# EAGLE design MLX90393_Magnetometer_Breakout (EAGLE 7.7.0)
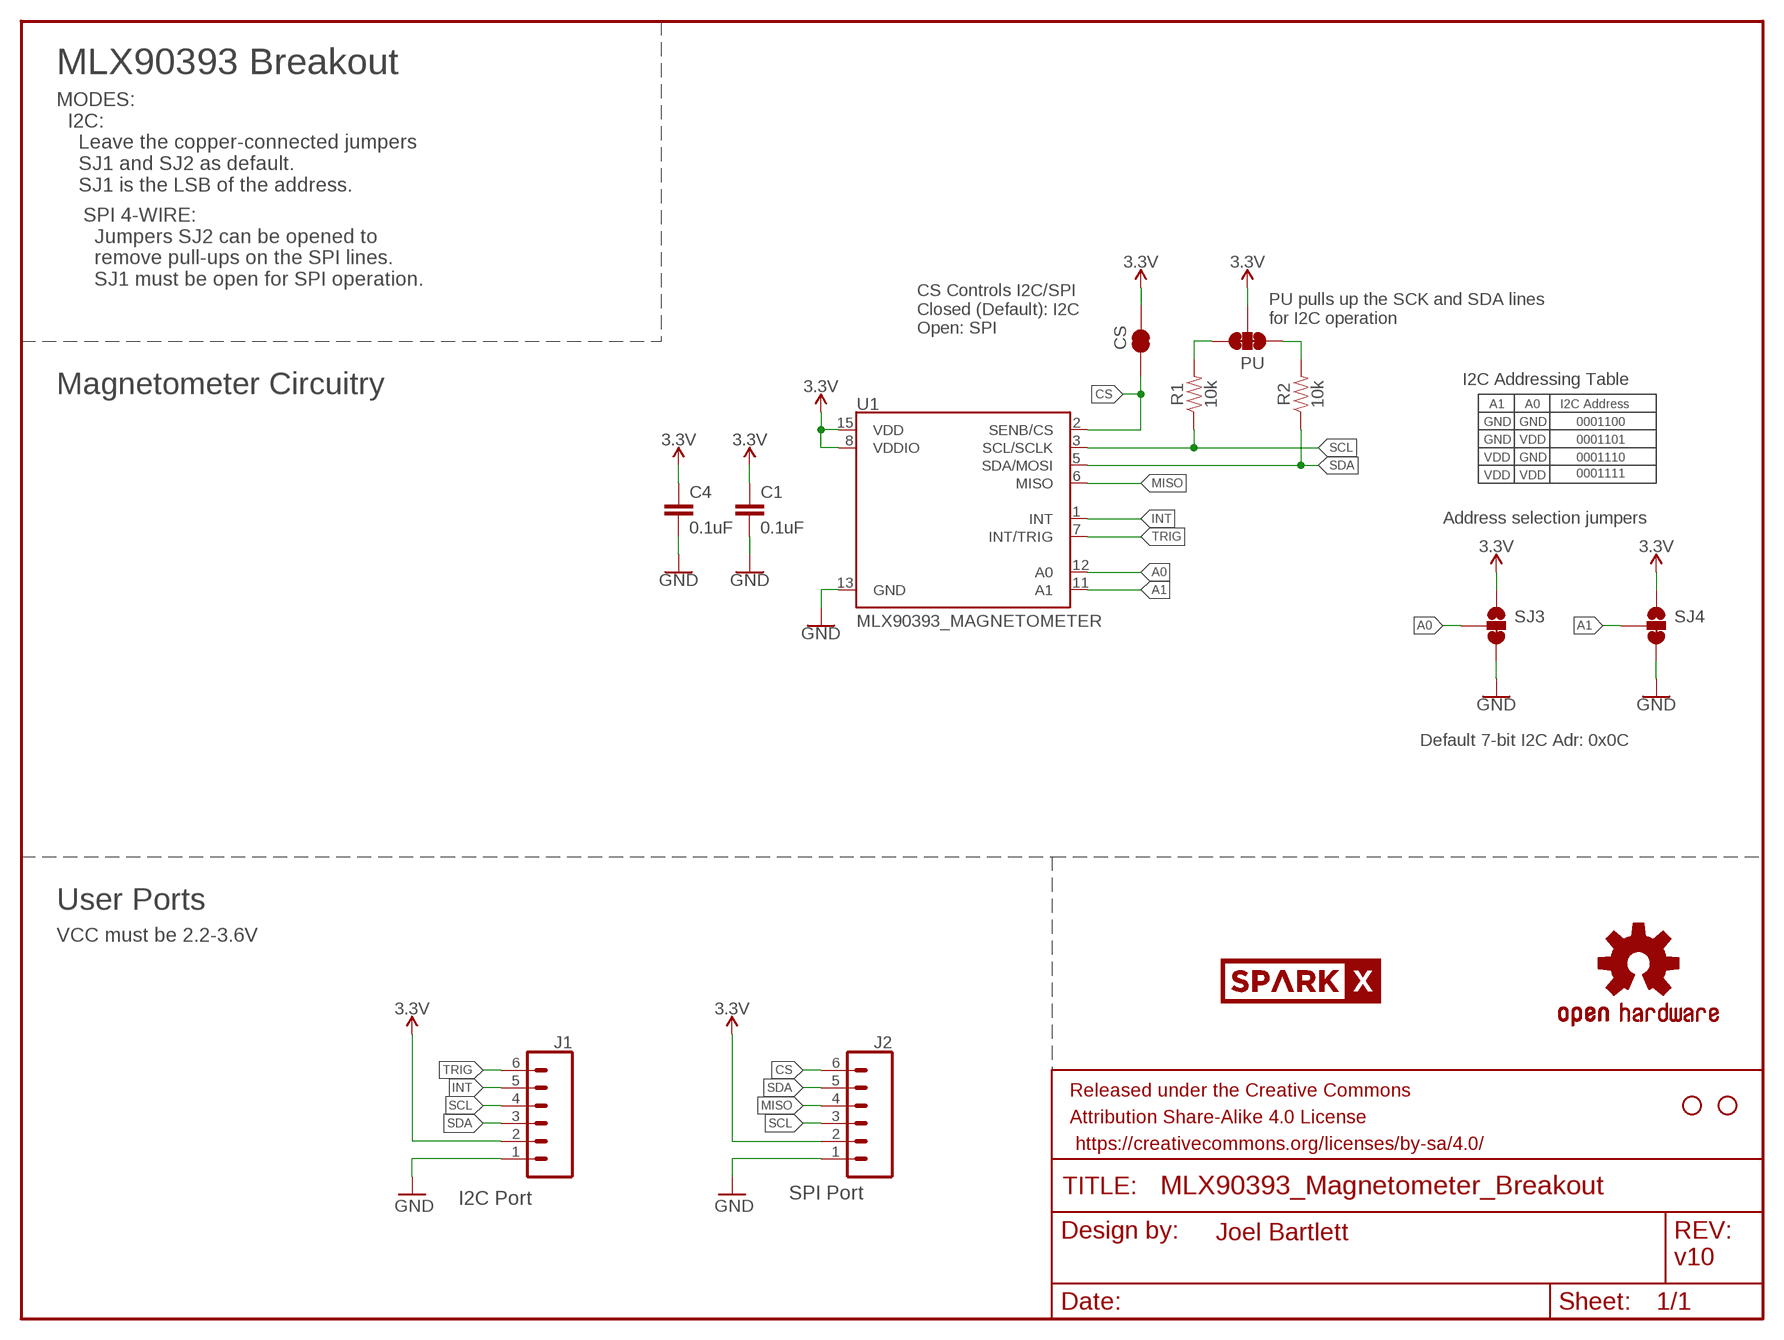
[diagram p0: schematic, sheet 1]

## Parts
C1  0.1uF  0.1UF-0603-25V-(+80/-20%)  [0603]
C4  0.1uF  0.1UF-0603-25V-(+80/-20%)  [0603]
CS  JUMPER-SMT_2_NC_TRACE_SILK  [SMT-JUMPER_2_NC_TRACE_SILK]
FRAME2  FRAME-LETTER  [CREATIVE_COMMONS]
J1  CONN_06NO_SILK_FEMALE_PTH  [1X06_NO_SILK]
J2  CONN_06NO_SILK_FEMALE_PTH  [1X06_NO_SILK]
JP3  STAND-OFF  [STAND-OFF]
JP4  STAND-OFF  [STAND-OFF]
PU  JUMPER-PAD-3-NC_BY_TRACE  [PAD-JUMPER-3-3OF3_NC_BY_TRACE_YES_SILK_FULL_BOX]
R1  10k  10KOHM-0603-1/10W-1%  [0603]
R2  10k  10KOHM-0603-1/10W-1%  [0603]
SJ3  JUMPER-SMT_3_1-NC_TRACE_SILK  [SMT-JUMPER_3_1-NC_TRACE_SILK]
SJ4  JUMPER-SMT_3_1-NC_TRACE_SILK  [SMT-JUMPER_3_1-NC_TRACE_SILK]
U1  MLX90393_MAGNETOMETER  [QFN-16]
U$1  OSHW-LOGOS  [OSHW-LOGO-S]
U$2  SPARKX-LOGO2  [SPARKX-TINY]

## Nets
3.3V: C1.1 C4.1 CS.2 J1.2 J2.2 PU.2 SJ3.1 SJ4.1 U1.8(VDDIO) U1.15(VDD)
A0: SJ3.2 U1.12(A0)
A1: SJ4.2 U1.11(A1)
CS: CS.1 J2.6 U1.2(SENB/CS)
GND: C1.2 C4.2 J1.1 J2.1 SJ3.3 SJ4.3 U1.13(GND)
INT: J1.5 U1.1(INT)
MISO: J2.4 U1.6(MISO)
N$4: PU.1 R2.2
N$5: PU.3 R1.2
SCL: J1.4 J2.3 R1.1 U1.3(SCL/SCLK)
SDA: J1.3 J2.5 R2.1 U1.5(SDA/MOSI)
TRIG: J1.6 U1.7(INT/TRIG)

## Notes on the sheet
- MLX90393 Breakout
- MODES:
    I2C:
      Leave the copper-connected jumpers
      SJ1 and SJ2 as default.
      SJ1 is the LSB of the address.
- SPI 4-WIRE:
    Jumpers SJ2 can be opened to 
    remove pull-ups on the SPI lines.
    SJ1 must be open for SPI operation.
- PU pulls up the SCK and SDA lines
  for I2C operation
- CS Controls I2C/SPI
  Closed (Default): I2C
  Open: SPI
- I2C Addressing Table
- Magnetometer Circuitry
- A1 | A0 | I2C Address
- GND | GND | 0001100
- GND | VDD | 0001101
- VDD | GND | 0001110
- VDD | VDD | 0001111
- Address selection jumpers
- Default 7-bit I2C Adr: 0x0C
- User Ports
- VCC must be 2.2-3.6V
- I2C Port | SPI Port
- Joel Bartlett
- v10

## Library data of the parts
C1 C4 = SparkFun-Capacitors:0.1UF: 0.1µF ceramic capacitors; PROD_ID: CAP-00810
CS = SparkFun-Jumpers:JUMPER-SMT_2_NC_TRACE: Normally closed trace jumper
FRAME2 = SparkFun-Aesthetics:FRAME-LETTER: Schematic Frame
J1 J2 = SparkFun-Connectors:CONN_06: Header 6 Standard 6-pin 0.1" header. Use with straight break away headers (SKU : PRT-00116), right angle break away headers (PRT-00553), swiss pins (PRT-00743), machine pins (PRT-00117), and female headers (PRT-00115). Molex polarized connector foot print use with SKU : PRT-08094 with associated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; PROD_ID: CONN-08437
JP3 JP4 = SparkFun:STAND-OFF: Stand Off
PU = TestAperatures:JUMPER-PAD-3-NC_BY_TRACE
R1 R2 = SparkFun-Resistors:10KOHM: 10kΩ resistor; PROD_ID: RES-00824
SJ3 SJ4 = SparkFun-Jumpers:JUMPER-SMT_3_1-NC_TRACE: Normally closed trace jumper (1 of 2 connections) This jumper has a trace between two pads so it's normally closed (NC). The other connection is normally open (NO). Use a razor knife to open the connection. For best results follow the IPC guidelines for cutting traces: Cutout at least 0.063 mm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
U1 = SparkX:MLX90393_MAGNETOMETER
U$1 = SparkFun:OSHW-LOGO: Open Source Hardware Logo This logo indicates the piece of hardware it is found on incorporates a OSHW license and/or adheres to the definition of open source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
U$2 = SparkX:SPARKX-LOGO

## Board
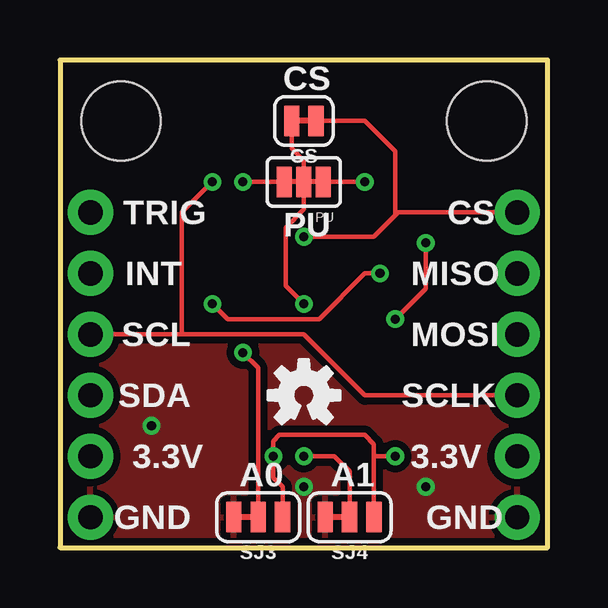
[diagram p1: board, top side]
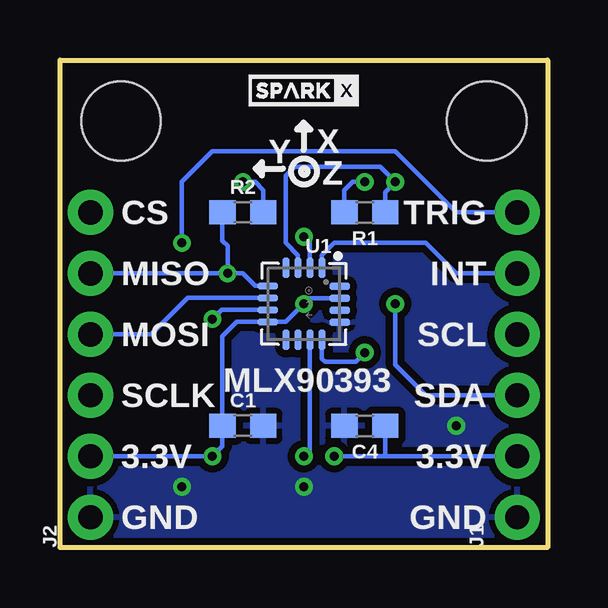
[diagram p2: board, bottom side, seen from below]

Size 20.32 x 20.32 mm. Coordinates in mm from the lower left corner, seen from the top.
Outline: 0,0 20.32,0 20.32,20.32 0,20.32 0,0
Copper layers (1*16): Top 0.035mm / dielectric 1.5mm / Bottom 0.035mm
Design rules "SparkFun-2-layer-TIGHT": minimum track width 7mil, minimum drill 15mil, track to track 7mil, track to pad 7mil, pad to pad 7mil, via to via 7mil, smd to smd 7mil, copper to edge 7mil, drill to drill 7mil, minimum pad ring 7mil, minimum via ring 7mil, stop-mask expansion 4mil, vias tented up to drill 25mil, thermal gap 10mil

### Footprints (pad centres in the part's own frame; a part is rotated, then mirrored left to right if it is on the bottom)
0603 = smd 1.1 x 1: 1 -0.85,0; 2 0.85,0
SMT-JUMPER_2_NC_TRACE_SILK = smd 0.635 x 1.27: 1 -0.508,0; 2 0.508,0
1X06_NO_SILK = drill 1.016 pad 1.88: 1 0,0; 2 2.54,0; 3 5.08,0; 4 7.62,0; 5 10.16,0; 6 12.7,0
STAND-OFF = hole 3.302: 0,0
PAD-JUMPER-3-3OF3_NC_BY_TRACE_YES_SILK_FULL_BOX = smd 0.635 x 1.27: 1 -0.813,0; 2 0,0; 3 0.813,0
SMT-JUMPER_3_1-NC_TRACE_SILK = smd 0.635 x 1.27: 1 -1.016,0; 2 0,0; 3 1.016,0
QFN-16 = smd 0.3 x 0.85: 1 0.754,1.498; 2 0.254,1.498; 3 -0.246,1.498; 4 -0.746,1.498; 9 -0.746,-1.506; 10 -0.246,-1.506; 11 0.254,-1.506; 12 0.754,-1.506 | smd 0.85 x 0.3: 5 -1.508,0.746; 6 -1.508,0.246; 7 -1.508,-0.254; 8 -1.508,-0.754; 13 1.496,-0.764; 14 1.496,-0.264; 15 1.496,0.236; 16 1.496,0.736

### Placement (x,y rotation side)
C1  12.7,5.08 0 bottom
C4  7.62,5.08 180 bottom
CS  10.16,17.78 180 top
FRAME2  not placed on the board
J1  1.27,1.27 90 bottom
J2  19.05,1.27 90 bottom
JP3  17.78,17.78 0 bottom
JP4  2.54,17.78 0 bottom
PU  10.16,15.24 180 top
R1  7.62,13.97 180 bottom
R2  12.7,13.97 0 bottom
SJ3  8.26,1.27 180 top
SJ4  12.06,1.27 180 top
U1  10.16,10.16 0 bottom
U$1  10.16,6.35 0 top
U$2  10.16,19.05 0 bottom

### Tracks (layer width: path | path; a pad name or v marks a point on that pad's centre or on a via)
3.3V  (via drill 0.38)
  Top 0.178: CS.2 9.65,16.64 10.16,16.13 PU.2 10.16,14.1 9.4,13.34 9.4,10.92 v10.16,10.16 | SJ4.1 13.08,3.81 | 13.08,3.81 13.08,4.32 12.7,4.7 9.14,4.7 8.89,4.45 v8.89,3.81 8.89,2.92 9.27,2.54 SJ3.1 | v13.97,3.81 13.08,3.81
  Bottom 0.178: U1.15 9.92,10.4 v10.16,10.16 10.91,9.41 U1.8 12.95,9.41 13.55,8.8 C1.1 13.55,4.23 v13.97,3.81 J2.2 | v8.89,3.81 6.86,3.81 | 6.86,3.81 J1.2 | C4.1 6.77,3.9 6.86,3.81
A0  (via drill 0.38)
  Top 0.178: SJ3.2 8.26,7.49 v7.62,8.13
  Bottom 0.178: U1.12 9.41,7.88 9.27,7.75 8,7.75 v7.62,8.13
A1  (via drill 0.38)
  Top 0.178: v10.16,3.81 11.43,3.81 12.06,3.17 SJ4.2
  Bottom 0.178: U1.11 9.91,4.06 v10.16,3.81
CS  (via drill 0.38)
  Top 0.178: CS.1 12.7,17.78 13.97,16.51 13.97,13.84 | v10.16,12.95 13.08,12.95 13.97,13.84 | J2.6 14.1,13.97 13.97,13.84
  Bottom 0.178: U1.2 9.91,12.7 v10.16,12.95
GND  (via drill 0.38)
  other vias: 15.24,2.54 10.16,2.54 3.81,5.08
  pour Bottom (isolate 0.305): 20.32,20.32 20.32,0 0,0 0,20.32
  pour Top (isolate 0.305): 20.32,20.32 20.32,0 0,0 0,20.32
INT
  Bottom 0.178: U1.1 9.41,12.18 8.89,12.7 5.08,12.7 3.81,11.43 J1.5
MISO
  Bottom 0.178: U1.6 14.99,10.41 16.51,8.89 J2.4
N$4  (via drill 0.38)
  Top 0.178: PU.1 v12.7,15.24
  Bottom 0.178: R2.2 11.85,14.9 12.19,15.24 v12.7,15.24
N$5  (via drill 0.38)
  Top 0.178: PU.3 v7.62,15.24
  Bottom 0.178: R1.2 8.47,14.9 8.13,15.24 v7.62,15.24
SCL  (via drill 0.38)
  Top 0.178: J2.3 12.7,6.35 10.16,8.89 5.08,8.89 | 5.08,8.89 J1.4 | v6.35,15.24 5.08,13.97 5.08,8.89
  Bottom 0.178: R1.1 6.77,14.82 v6.35,15.24 6.98,15.88 10.54,15.88 10.92,15.49 10.92,12.7 10.41,12.18 U1.3
SDA  (via drill 0.38)
  Top 0.178: v6.35,10.16 6.98,9.53 10.79,9.53 12.7,11.43 v13.34,11.43
  Bottom 0.178: U1.5 12.18,10.91 12.7,11.43 v13.34,11.43 | J1.3 5.08,6.35 6.35,7.62 v6.35,10.16 | R2.1 13.55,12.79 13.34,12.57 v13.34,11.43 | v13.34,11.43 J2.5
TRIG  (via drill 0.38)
  Top 0.178: v15.24,12.7 15.24,10.79 v13.97,9.53
  Bottom 0.178: U1.7 13.59,9.91 v13.97,9.53 | J1.6 3.81,13.97 6.35,16.51 13.97,16.51 15.24,15.24 v15.24,12.7

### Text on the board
tPlace: CS | TRIG | PU | CS | INT | MISO | SCL | MOSI | SDA | SCLK | 3.3V | A0 | A1 | 3.3V | GND | GND
bPlace: X | Y | Z | TRIG | CS | INT | MISO | SCL | MOSI | MLX90393 | SDA | SCLK | 3.3V | 3.3V | GND | GND
bDocu: J. Bartlett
